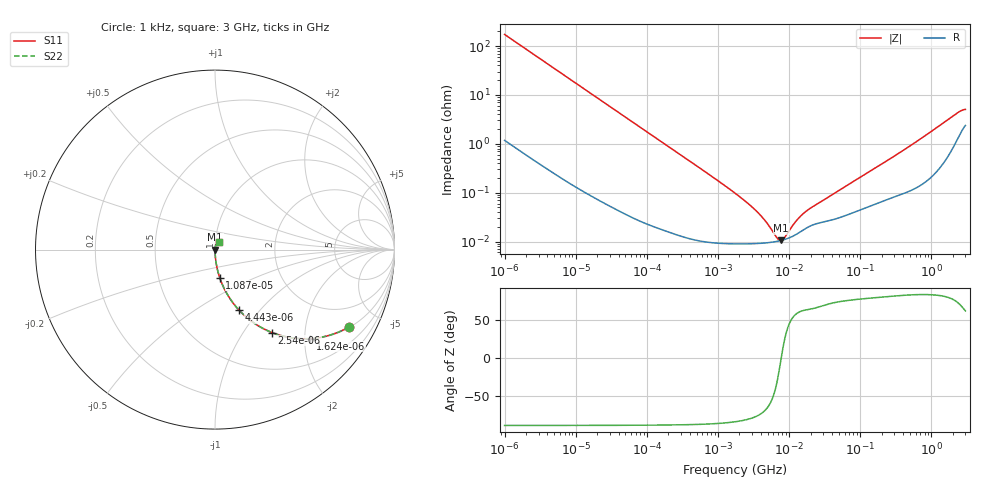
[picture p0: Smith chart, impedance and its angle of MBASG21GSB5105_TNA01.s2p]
! MBASG21GSB5105_TNA01  S-PARAMETER MODEL  ( Standard Model )
! Model Generated by TAIYO YUDEN Corporation (http://www.ty-top.com)
! Version 1.0
! TAIYO YUDEN Control No. 220601
! Copyright(c) 2012 TAIYO YUDEN CO.,LTD. All Rights Reserved.
! Product Description (link to TY-COMPAS)
! https://ds.yuden.co.jp/TYCOMPAS/or/detail?pn=MBASG21GSB5105KTNA01&u=M
! Products Name : Multilayer Ceramic Capacitors
! Characteristics :
!  Capacitance : 1 [uF] , Rated Voltage : 35 [V] , TCC : X5R
!  Case Size : 2.0 x 1.25 / 0.079 x 0.049 [mm/inch] , Thickness : 1.25 / 0.049 [mm/inch]
!  (Conditions: Temperature = 25 [degC] , DC Bias Voltage = 0 [V])
! External Node Assignments :
!  1  o---| |---o  2
! GND o---------o GND
! Frequency Range : 1kHz  -  3GHz  [ 401 STEP ]
# MHZ S RI R 50
! Freq[MHz].  S11 Real  S11 Imag  S21 Real  S21 Imag  S12 Real  S12 Imag  S22 Real  S22 Imag
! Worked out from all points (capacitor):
!   401 points, 1 kHz to 3 GHz, reference 50 ohm
!   read as one part in series: C = 921 nF near 1.077 kHz
!   lowest |Z| = 10.5 mohm at 7.696 MHz (marker M1)
!   series resonance near 7.746 MHz, so ESL is about 460 pH
!   S11 on the Smith chart (normalised r, x): 1 kHz: 1.02, -3.45; 1.624 kHz: 1.01, -2.13; 2.54 kHz: 1.01, -1.36; 4.443 kHz: 1.01, -0.78; 10.87 kHz: 1.00, -0.32; 3 GHz: 1.05, +0.09
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0.001  0.747 -0.4314  0.253 0.4314  0.253 0.4314  0.747 -0.4314
0.001624  0.531 -0.4957  0.469 0.4957  0.469 0.4957  0.531 -0.4957
0.00254  0.3185 -0.4625  0.6815 0.4625  0.6815 0.4625  0.3185 -0.4625
0.004443  0.1342 -0.3373  0.8658 0.3373  0.8658 0.3373  0.1342 -0.3373
0.006696  0.0647 -0.2424  0.9353 0.2424  0.9353 0.2424  0.0647 -0.2424
0.010873  0.0262 -0.1559  0.9738 0.1559  0.9738 0.1559  0.0262 -0.1559
0.01216  0.0212 -0.1402  0.9788 0.1402  0.9788 0.1402  0.0212 -0.1402
0.033275  0.00325 -0.0524  0.9968 0.0524  0.9968 0.0524  0.00325 -0.0524
0.147855  0.000326 -0.0119  0.9997 0.0119  0.9997 0.0119  0.000326 -0.0119
1.732051  9.06e-05 -0.000976  0.9999 0.000976  0.9999 0.000976  9.06e-05 -0.000976
3.651041  9.16e-05 -0.000379  0.9999 0.000379  0.9999 0.000379  9.16e-05 -0.000379
4.739869  9.41e-05 -0.000235  0.9999 0.000235  0.9999 0.000235  9.41e-05 -0.000235
6.629817  0.0001 -7.15e-05  0.9999 7.15e-05  0.9999 7.15e-05  0.0001 -7.15e-05
7.143107  0.000103 -3.71e-05  0.9999 3.71e-05  0.9999 3.71e-05  0.000103 -3.71e-05
7.696136  0.000105 -2.93e-06  0.9999 2.93e-06  0.9999 2.93e-06  0.000105 -2.93e-06
8.606987  0.00011 4.82e-05  0.9999 -4.82e-05  0.9999 -4.82e-05  0.00011 4.82e-05
11.59828  0.000132 0.000187  0.9999 -0.000187  0.9999 -0.000187  0.000132 0.000187
13.97519  0.000154 0.000275  0.9998 -0.000275  0.9998 -0.000275  0.000154 0.000275
21.06097  0.000217 0.000461  0.9998 -0.000461  0.9998 -0.000461  0.000217 0.000461
256.0921  0.000773 0.00477  0.9992 -0.00477  0.9992 -0.00477  0.000773 0.00477
2226.275  0.0124 0.039  0.9876 -0.039  0.9876 -0.039  0.0124 0.039
3000  0.025 0.0425  0.975 -0.0425  0.975 -0.0425  0.025 0.0425
